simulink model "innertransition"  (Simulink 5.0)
settings: Solver=ode1  StartTime=0.0  StopTime=100  FixedStep=0.0001  RelTol=1e-3
libraries: simulink x1

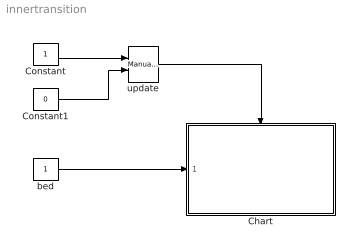
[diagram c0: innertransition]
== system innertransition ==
  Chart : Stateflow chart  TreatAsAtomicUnit=on
  Constant : Constant
  Constant1 : Constant  Value=0
  bed : Constant
  update : simulink/Signal Routing/Manual Switch  sw=0  action=0
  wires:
  Constant1/1 -> update/2
  Constant/1 -> update/1
  update/1 -> Chart/Trigger
  bed/1 -> Chart/1(bed)

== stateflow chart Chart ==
  state Super_Z
    state Z1
    state Z2
    state Z3
    Super_Z -> (junction 7) : update
    (default) -> (junction 7)
    (junction 7) -> Z1 : [bed==1]
    (junction 7) -> Z2 : [bed==2]
    (junction 7) -> Z3
